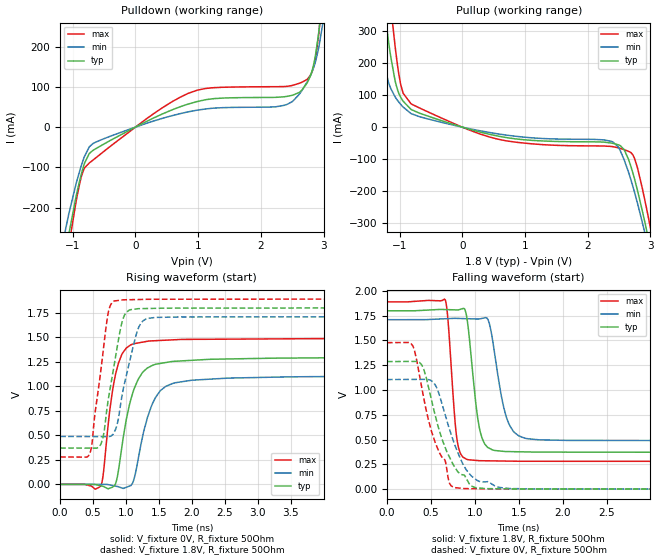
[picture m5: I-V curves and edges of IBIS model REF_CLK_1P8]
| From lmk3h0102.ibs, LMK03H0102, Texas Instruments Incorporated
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[Model]   REF_CLK_1P8
Model_type   Output
Polarity   Non-Inverting
Vmeas = 0.9
Vref = 0
Cref = 5pF
Rref = 100000
|   typ   min   max
C_comp   2.5pF   2pF   3pF
[Voltage Range]   1.8   1.71   1.89
[Temperature Range]   45   125   -40
[Pullup Reference]   1.8   1.71   1.89
[Pulldown Reference]   0   0   0
[Power Clamp Reference]   1.8   1.71   1.89
[GND Clamp Reference]   0   0   0
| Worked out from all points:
|   slope of the pulldown table from 0 to 0.27 V, typ, clamps not added: 12.7 ohm
|   slope of the pullup table from 0 to 0.27 V, typ, clamps not added: 18.4 ohm
|   falling waveform, V_fixture 1.8V, R_fixture 50Ohm: 20-80 % time 106ps typ, 148ps min, 76.9ps max; typ from 1.8 V to 0.371 V
|   rising waveform, V_fixture 0V, R_fixture 50Ohm: 20-80 % time 251ps typ, 272ps min, 184ps max; typ from 0 V to 1.29 V
|   rising waveform, V_fixture 1.8V, R_fixture 50Ohm: 20-80 % time 206ps typ, 231ps min, 180ps max; typ from 0.371 V to 1.8 V
|   falling waveform, V_fixture 0V, R_fixture 50Ohm: 20-80 % time 275ps typ, 266ps min, 294ps max; typ from 1.29 V to 0 V
[Pulldown]
|   Voltage   I(typ)   I(min)   I(max)
-3.3V     -2.545A    -2.251A    -2.867A
-1.221V   -401.9mA   -333.2mA   -455.9mA
-1.063V   -267.1mA   -216mA     -295.7mA
-815.1mV  -90.95mA   -73.76mA   -101.8mA
-676.5mV  -57.76mA   -40.74mA   -81.81mA
848.1mV   57.63mA    38.18mA    84.24mA
2.422V    76.58mA    56.88mA    101.4mA
2.788V    126.5mA    127.3mA    128.5mA
2.858V    167.6mA    155.6mA    160.7mA
2.927V    239.8mA    200.8mA    237.5mA
2.986V    321.6mA    256.3mA    333.5mA
6.6V      7.419A     6.213A     8.998A
[Pullup]
|   Voltage   I(typ)   I(min)   I(max)
-3.3V     4.353A     3.467A     5.481A
-1.409V   653.7mA    386.6mA    939.4mA
-1.28V    430mA      228.3mA    659.8mA
-1.142V   221.6mA    121.5mA    380.1mA
-983.4mV  93.69mA    71.53mA    134.9mA
-815.1mV  55.18mA    42.23mA    72.62mA
590.7mV   -28.77mA   -21.73mA   -38.71mA
2.402V    -50.85mA   -46.4mA    -61.2mA
2.719V    -142.9mA   -184.8mA   -86.63mA
2.917V    -303mA     -336.2mA   -234.5mA
3.066V    -441.6mA   -461.3mA   -378.5mA
6.6V      -4.064A    -3.692A    -4.487A
[Ramp]
R_load = 50
|   typ   min   max
dV/dt_r   0.776784/2.48605e-10   0.662987/2.71462e-10   0.894124/1.82887e-10
dV/dt_f   0.85746/1.04822e-10   0.732787/1.47985e-10   0.966203/7.69065e-11
[Falling Waveform]
V_fixture = 1.8V
V_fixture_min = 1.71V
V_fixture_max = 1.89V
R_fixture = 50Ohm
C_fixture = 0F
|   Time   V(typ)   V(min)   V(max)
0s        1.8V       1.71V      1.89V
661.7ps   1.812V     1.719V     1.91V
694.1ps   1.811V     1.721V     1.691V
790.7ps   1.809V     1.723V     530.9mV
904.6ps   1.744V     1.72V      301.4mV
1.049ns   621.4mV    1.717V     287.3mV
1.197ns   396.7mV    1.52V      285.5mV
1.359ns   379.6mV    720.3mV    283.5mV
1.56ns    376.3mV    516.1mV    281.7mV
5ns       370.9mV    488.7mV    279.6mV
[Rising Waveform]
V_fixture = 0V
V_fixture_min = 0V
V_fixture_max = 0V
R_fixture = 50Ohm
C_fixture = 0F
|   Time   V(typ)   V(min)   V(max)
0s        798.7nV    2.602uV    692.4nV
618.6ps   -14.71mV   -307.2uV   -13.37mV
758.1ps   -37.78mV   -6.565mV   777.8mV
836.7ps   1.064mV    -17.16mV   1.107V
934.8ps   370.5mV    -36.25mV   1.322V
1.071ns   860.5mV    -12.95mV   1.422V
1.182ns   1.068V     246.8mV    1.442V
1.382ns   1.207V     791.6mV    1.463V
1.697ns   1.253V     1.027V     1.474V
5ns       1.295V     1.105V     1.49V
[Rising Waveform]
V_fixture = 1.8V
V_fixture_min = 1.71V
V_fixture_max = 1.89V
R_fixture = 50Ohm
C_fixture = 0F
|   Time   V(typ)   V(min)   V(max)
0s        370.7mV    488.4mV    279.5mV
455.7ps   369.7mV    487.6mV    325.6mV
642.3ps   456.7mV    487.3mV    1.297V
736.8ps   889.7mV    487.1mV    1.771V
815.5ps   1.2V       525.2mV    1.868V
876.8ps   1.442V     645mV      1.875V
981.3ps   1.731V     1.041V     1.883V
1.168ns   1.79V      1.556V     1.885V
1.308ns   1.793V     1.688V     1.887V
5ns       1.8V       1.71V      1.89V
[Falling Waveform]
|Gnd
V_fixture = 0V
V_fixture_min = 0V
V_fixture_max = 0V
R_fixture = 50Ohm
C_fixture = 0F
|   Time   V(typ)   V(min)   V(max)
0s        1.287V     1.106V     1.478V
293.6ps   1.289V     1.107V     1.444V
417.6ps   1.209V     1.108V     918.3mV
532.5ps   797.8mV    1.072V     511mV
625.7ps   502.5mV    857.1mV    320mV
708ps     326.6mV    609.1mV    64.8mV
758.1ps   239.9mV    475.1mV    18.28mV
956.6ps   34.05mV    134.3mV    5.068mV
1.283ns   3.94mV     16.9mV     1.719mV
5ns       109.6uV    161.7uV    69.32uV
